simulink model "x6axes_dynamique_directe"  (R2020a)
settings: Solver=VariableStepAuto  StartTime=0.0  StopTime=t(numel(t))  FixedStep=dt  RelTol=1e-3
model workspace: external: MATLAB File (data not in the file)
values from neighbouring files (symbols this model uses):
  D = [10 10 10 0 0 0]    [TP_6Axes_main.m]
  mu = mu/3    [TP_6Axes_main.m]
  P = [10000 10000 10000 1000 1000 1000]    [TP_6Axes_main.m]
  q_targ = zeros(6,numel(X(1,:)))    [TP_6axes_trajectoire_rectangulaire_min_jerk.m]
  X = [X1(:,1:numel(X1(1,:))-1) X2]    [concat_motion.m]    (also in MGD_6axes.m = [T(1:3,4);Euler]; Trace_6axes.m = [0 0 0; Trace_6axes_trajectoire.m = [0 0 0)
undefined symbols (not defined in the file or in its folder): deg, kg, m, mm, N, rad, s, smiData, Y, Z
libraries: sm_lib x37, nesl_utility x22

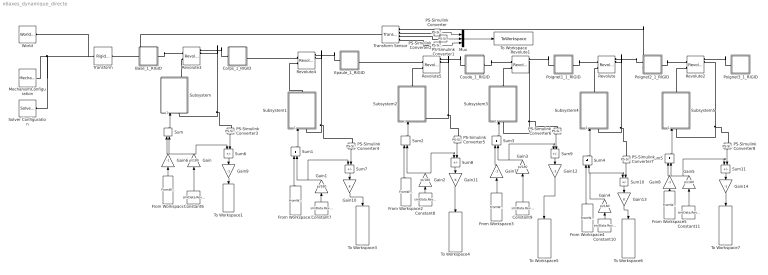
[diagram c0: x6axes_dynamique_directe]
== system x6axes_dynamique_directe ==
  Base_1_RIGID : Subsystem
  Constant10 : Constant  Value=smiData.RevoluteJoint(1).Rz.Pos
  Constant11 : Constant  Value=smiData.RevoluteJoint(3).Rz.Pos
  Constant6 : Constant  Value=smiData.RevoluteJoint(4).Rz.Pos
  Constant7 : Constant  Value=smiData.RevoluteJoint(5).Rz.Pos
  Constant8 : Constant  Value=smiData.RevoluteJoint(6).Rz.Pos
  Constant9 : Constant  Value=smiData.RevoluteJoint(2).Rz.Pos
  Corps_1_RIGID : Subsystem
  Coude_1_RIGID : Subsystem
  Epaule_1_RIGID : Subsystem
  From Workspace : FromWorkspace  VariableName=[t' q_targ(1,:)']
  From Workspace1 : FromWorkspace  VariableName=[t' q_targ(2,:)']
  From Workspace2 : FromWorkspace  VariableName=[t' q_targ(3,:)']
  From Workspace3 : FromWorkspace  VariableName=[t' q_targ(4,:)']
  From Workspace4 : FromWorkspace  VariableName=[t' q_targ(5,:)']
  From Workspace5 : FromWorkspace  VariableName=[t' q_targ(6,:)']
  Gain{,1..5} (6 alike) : Gain  Gain=pi/180
  Gain10 : Gain
  Gain11 : Gain
  Gain{6..9,12,14} (6 alike) : Gain  Gain=-1
  Gain13 : Gain
  MechanismConfiguration : sm_lib/Utilities/Mechanism Configuration  UniformGravity=Constant  GravityVector=[0 0 -9.80665]  GravityUnits=m/s^2  LinearizationDelta=0.001
  Mux : Mux  Inputs=3
  PS-Simulink Converter : nesl_utility/PS-Simulink Converter  PhysicalDomain=network_engine_domain  SubClassName=ps_output  LeftPortType=input  RightPortType=output  PseudoPeriodic=off  Frequencies=[]  Unit=m  AffineConversion=off
  PS-Simulink Converter1 : nesl_utility/PS-Simulink Converter  PhysicalDomain=network_engine_domain  SubClassName=ps_output  LeftPortType=input  RightPortType=output  PseudoPeriodic=off  Frequencies=[]  Unit=m  AffineConversion=off
  PS-Simulink Converter2 : nesl_utility/PS-Simulink Converter  PhysicalDomain=network_engine_domain  SubClassName=ps_output  LeftPortType=input  RightPortType=output  PseudoPeriodic=off  Frequencies=[]  Unit=m  AffineConversion=off
  PS-Simulink Converter{3..8} (6 alike) : nesl_utility/PS-Simulink Converter  PhysicalDomain=network_engine_domain  SubClassName=ps_output  LeftPortType=input  RightPortType=output  PseudoPeriodic=off  Frequencies=[]  Unit=rad  AffineConversion=off
  Poignet1_1_RIGID : Subsystem
  Poignet2_1_RIGID : Subsystem
  Poignet3_1_RIGID : Subsystem
  Revolute : sm_lib/Joints/Revolute Joint  JointMode=Normal  SenseConstraintForce=off  SenseConstraintForceX=off  SenseConstraintForceY=off  SenseConstraintForceZ=off  SenseConstraintTorque=off  SenseConstraintTorqueX=off  SenseConstraintTorqueY=off  SenseConstraintTorqueZ=off  SenseTotalForce=off  SenseTotalForceX=off  SenseTotalForceY=off  SenseTotalForceZ=off  SenseTotalTorque=off  SenseTotalTorqueX=off  SenseTotalTorqueY=off  SenseTotalTorqueZ=off  CompositeWrenchDir=FollowerOnBase  CompositeWrenchFrame=BaseFrame  EquilibriumPosition=0  EquilibriumPositionUnits=rad  SpringStiffness=0  SpringStiffnessUnits=N*m/rad  DampingCoefficient=mu(5)  DampingCoefficientUnits=N*m/(rad/s)  TorqueActuationMode=InputTorque  MotionActuationMode=ComputedMotion  SensePosition=on  SenseVelocity=on  SenseAcceleration=on  SenseTorqueForce=on  SenseLowerLimitTorqueForce=off  SenseUpperLimitTorqueForce=off  LowerLimitSpecify=off  LowerLimitBound=-90  LowerLimitBoundUnits=deg  LowerLimitStiffness=1e4  LowerLimitStiffnessUnits=N*m/deg  LowerLimitDamping=10  LowerLimitDampingUnits=N*m/(deg/s)  LowerLimitTransitionRegionWidth=0.1  LowerLimitTransitionRegionWidthUnits=deg  UpperLimitSpecify=off  UpperLimitBound=90  UpperLimitBoundUnits=deg  UpperLimitStiffness=1e4  UpperLimitStiffnessUnits=N*m/deg  UpperLimitDamping=10  UpperLimitDampingUnits=N*m/(deg/s)  UpperLimitTransitionRegionWidth=0.1  UpperLimitTransitionRegionWidthUnits=deg  PositionTargetSpecify=on  PositionTargetPriority=Low  PositionTargetValue=smiData.RevoluteJoint(1).Rz.Pos*pi/180+q_targ(5,1)  PositionTargetValueUnits=rad  VelocityTargetSpecify=on  VelocityTargetPriority=High  VelocityTargetValue=0  VelocityTargetValueUnits=deg/s
  Revolute1 : sm_lib/Joints/Revolute Joint  JointMode=Normal  SenseConstraintForce=off  SenseConstraintForceX=off  SenseConstraintForceY=off  SenseConstraintForceZ=off  SenseConstraintTorque=off  SenseConstraintTorqueX=off  SenseConstraintTorqueY=off  SenseConstraintTorqueZ=off  SenseTotalForce=off  SenseTotalForceX=off  SenseTotalForceY=off  SenseTotalForceZ=off  SenseTotalTorque=off  SenseTotalTorqueX=off  SenseTotalTorqueY=off  SenseTotalTorqueZ=off  CompositeWrenchDir=FollowerOnBase  CompositeWrenchFrame=BaseFrame  EquilibriumPosition=0  EquilibriumPositionUnits=rad  SpringStiffness=0  SpringStiffnessUnits=N*m/rad  DampingCoefficient=mu(4)  DampingCoefficientUnits=N*m/(rad/s)  TorqueActuationMode=InputTorque  MotionActuationMode=ComputedMotion  SensePosition=on  SenseVelocity=on  SenseAcceleration=on  SenseTorqueForce=on  SenseLowerLimitTorqueForce=off  SenseUpperLimitTorqueForce=off  LowerLimitSpecify=off  LowerLimitBound=-90  LowerLimitBoundUnits=deg  LowerLimitStiffness=1e4  LowerLimitStiffnessUnits=N*m/deg  LowerLimitDamping=10  LowerLimitDampingUnits=N*m/(deg/s)  LowerLimitTransitionRegionWidth=0.1  LowerLimitTransitionRegionWidthUnits=deg  UpperLimitSpecify=off  UpperLimitBound=90  UpperLimitBoundUnits=deg  UpperLimitStiffness=1e4  UpperLimitStiffnessUnits=N*m/deg  UpperLimitDamping=10  UpperLimitDampingUnits=N*m/(deg/s)  UpperLimitTransitionRegionWidth=0.1  UpperLimitTransitionRegionWidthUnits=deg  PositionTargetSpecify=on  PositionTargetPriority=High  PositionTargetValue=smiData.RevoluteJoint(2).Rz.Pos*pi/180-q_targ(4,1)  PositionTargetValueUnits=rad  VelocityTargetSpecify=on  VelocityTargetPriority=High  VelocityTargetValue=0  VelocityTargetValueUnits=deg/s
  Revolute2 : sm_lib/Joints/Revolute Joint  JointMode=Normal  SenseConstraintForce=off  SenseConstraintForceX=off  SenseConstraintForceY=off  SenseConstraintForceZ=off  SenseConstraintTorque=off  SenseConstraintTorqueX=off  SenseConstraintTorqueY=off  SenseConstraintTorqueZ=off  SenseTotalForce=off  SenseTotalForceX=off  SenseTotalForceY=off  SenseTotalForceZ=off  SenseTotalTorque=off  SenseTotalTorqueX=off  SenseTotalTorqueY=off  SenseTotalTorqueZ=off  CompositeWrenchDir=FollowerOnBase  CompositeWrenchFrame=BaseFrame  EquilibriumPosition=0  EquilibriumPositionUnits=rad  SpringStiffness=0  SpringStiffnessUnits=N*m/rad  DampingCoefficient=mu(6)  DampingCoefficientUnits=N*m/(rad/s)  TorqueActuationMode=InputTorque  MotionActuationMode=ComputedMotion  SensePosition=on  SenseVelocity=on  SenseAcceleration=on  SenseTorqueForce=on  SenseLowerLimitTorqueForce=off  SenseUpperLimitTorqueForce=off  LowerLimitSpecify=off  LowerLimitBound=-90  LowerLimitBoundUnits=deg  LowerLimitStiffness=1e4  LowerLimitStiffnessUnits=N*m/deg  LowerLimitDamping=10  LowerLimitDampingUnits=N*m/(deg/s)  LowerLimitTransitionRegionWidth=0.1  LowerLimitTransitionRegionWidthUnits=deg  UpperLimitSpecify=off  UpperLimitBound=90  UpperLimitBoundUnits=deg  UpperLimitStiffness=1e4  UpperLimitStiffnessUnits=N*m/deg  UpperLimitDamping=10  UpperLimitDampingUnits=N*m/(deg/s)  UpperLimitTransitionRegionWidth=0.1  UpperLimitTransitionRegionWidthUnits=deg  PositionTargetSpecify=on  PositionTargetPriority=Low  PositionTargetValue=smiData.RevoluteJoint(3).Rz.Pos*pi/180-q_targ(6,1)  PositionTargetValueUnits=rad  VelocityTargetSpecify=on  VelocityTargetPriority=High  VelocityTargetValue=0  VelocityTargetValueUnits=deg/s
  Revolute3 : sm_lib/Joints/Revolute Joint  JointMode=Normal  SenseConstraintForce=off  SenseConstraintForceX=off  SenseConstraintForceY=off  SenseConstraintForceZ=off  SenseConstraintTorque=off  SenseConstraintTorqueX=off  SenseConstraintTorqueY=off  SenseConstraintTorqueZ=off  SenseTotalForce=off  SenseTotalForceX=off  SenseTotalForceY=off  SenseTotalForceZ=off  SenseTotalTorque=off  SenseTotalTorqueX=off  SenseTotalTorqueY=off  SenseTotalTorqueZ=off  CompositeWrenchDir=FollowerOnBase  CompositeWrenchFrame=BaseFrame  EquilibriumPosition=0  EquilibriumPositionUnits=rad  SpringStiffness=0  SpringStiffnessUnits=N*m/rad  DampingCoefficient=mu(1)  DampingCoefficientUnits=N*m/(rad/s)  TorqueActuationMode=InputTorque  MotionActuationMode=ComputedMotion  SensePosition=on  SenseVelocity=on  SenseAcceleration=on  SenseTorqueForce=on  SenseLowerLimitTorqueForce=off  SenseUpperLimitTorqueForce=off  LowerLimitSpecify=off  LowerLimitBound=-90  LowerLimitBoundUnits=deg  LowerLimitStiffness=1e4  LowerLimitStiffnessUnits=N*m/deg  LowerLimitDamping=10  LowerLimitDampingUnits=N*m/(deg/s)  LowerLimitTransitionRegionWidth=0.1  LowerLimitTransitionRegionWidthUnits=deg  UpperLimitSpecify=off  UpperLimitBound=90  UpperLimitBoundUnits=deg  UpperLimitStiffness=1e4  UpperLimitStiffnessUnits=N*m/deg  UpperLimitDamping=10  UpperLimitDampingUnits=N*m/(deg/s)  UpperLimitTransitionRegionWidth=0.1  UpperLimitTransitionRegionWidthUnits=deg  PositionTargetSpecify=on  PositionTargetPriority=High  PositionTargetValue=smiData.RevoluteJoint(4).Rz.Pos*pi/180-q_targ(1,1)  PositionTargetValueUnits=rad  VelocityTargetSpecify=on  VelocityTargetPriority=High  VelocityTargetValue=0  VelocityTargetValueUnits=deg/s
  Revolute4 : sm_lib/Joints/Revolute Joint  JointMode=Normal  SenseConstraintForce=off  SenseConstraintForceX=off  SenseConstraintForceY=off  SenseConstraintForceZ=off  SenseConstraintTorque=off  SenseConstraintTorqueX=off  SenseConstraintTorqueY=off  SenseConstraintTorqueZ=off  SenseTotalForce=off  SenseTotalForceX=off  SenseTotalForceY=off  SenseTotalForceZ=off  SenseTotalTorque=off  SenseTotalTorqueX=off  SenseTotalTorqueY=off  SenseTotalTorqueZ=off  CompositeWrenchDir=FollowerOnBase  CompositeWrenchFrame=BaseFrame  EquilibriumPosition=0  EquilibriumPositionUnits=rad  SpringStiffness=0  SpringStiffnessUnits=N*m/rad  DampingCoefficient=mu(2)  DampingCoefficientUnits=N*m/(rad/s)  TorqueActuationMode=InputTorque  MotionActuationMode=ComputedMotion  SensePosition=on  SenseVelocity=on  SenseAcceleration=on  SenseTorqueForce=on  SenseLowerLimitTorqueForce=off  SenseUpperLimitTorqueForce=off  LowerLimitSpecify=off  LowerLimitBound=-90  LowerLimitBoundUnits=deg  LowerLimitStiffness=1e4  LowerLimitStiffnessUnits=N*m/deg  LowerLimitDamping=10  LowerLimitDampingUnits=N*m/(deg/s)  LowerLimitTransitionRegionWidth=0.1  LowerLimitTransitionRegionWidthUnits=deg  UpperLimitSpecify=off  UpperLimitBound=90  UpperLimitBoundUnits=deg  UpperLimitStiffness=1e4  UpperLimitStiffnessUnits=N*m/deg  UpperLimitDamping=10  UpperLimitDampingUnits=N*m/(deg/s)  UpperLimitTransitionRegionWidth=0.1  UpperLimitTransitionRegionWidthUnits=deg  PositionTargetSpecify=on  PositionTargetPriority=High  PositionTargetValue=smiData.RevoluteJoint(5).Rz.Pos*pi/180+q_targ(2,1)  PositionTargetValueUnits=rad  VelocityTargetSpecify=on  VelocityTargetPriority=High  VelocityTargetValue=0  VelocityTargetValueUnits=deg/s
  Revolute5 : sm_lib/Joints/Revolute Joint  JointMode=Normal  SenseConstraintForce=off  SenseConstraintForceX=off  SenseConstraintForceY=off  SenseConstraintForceZ=off  SenseConstraintTorque=off  SenseConstraintTorqueX=off  SenseConstraintTorqueY=off  SenseConstraintTorqueZ=off  SenseTotalForce=off  SenseTotalForceX=off  SenseTotalForceY=off  SenseTotalForceZ=off  SenseTotalTorque=off  SenseTotalTorqueX=off  SenseTotalTorqueY=off  SenseTotalTorqueZ=off  CompositeWrenchDir=FollowerOnBase  CompositeWrenchFrame=BaseFrame  EquilibriumPosition=0  EquilibriumPositionUnits=rad  SpringStiffness=0  SpringStiffnessUnits=N*m/rad  DampingCoefficient=mu(3)  DampingCoefficientUnits=N*m/(rad/s)  TorqueActuationMode=InputTorque  MotionActuationMode=ComputedMotion  SensePosition=on  SenseVelocity=on  SenseAcceleration=on  SenseTorqueForce=on  SenseLowerLimitTorqueForce=off  SenseUpperLimitTorqueForce=off  LowerLimitSpecify=off  LowerLimitBound=-90  LowerLimitBoundUnits=deg  LowerLimitStiffness=1e4  LowerLimitStiffnessUnits=N*m/deg  LowerLimitDamping=10  LowerLimitDampingUnits=N*m/(deg/s)  LowerLimitTransitionRegionWidth=0.1  LowerLimitTransitionRegionWidthUnits=deg  UpperLimitSpecify=off  UpperLimitBound=90  UpperLimitBoundUnits=deg  UpperLimitStiffness=1e4  UpperLimitStiffnessUnits=N*m/deg  UpperLimitDamping=10  UpperLimitDampingUnits=N*m/(deg/s)  UpperLimitTransitionRegionWidth=0.1  UpperLimitTransitionRegionWidthUnits=deg  PositionTargetSpecify=on  PositionTargetPriority=High  PositionTargetValue=smiData.RevoluteJoint(6).Rz.Pos*pi/180+q_targ(3,1)  PositionTargetValueUnits=rad  VelocityTargetSpecify=on  VelocityTargetPriority=High  VelocityTargetValue=0  VelocityTargetValueUnits=deg/s
  Solver Configuration : nesl_utility/Solver Configuration  PhysicalDomain=network_engine_domain  SubClassName=solver  LeftPortType=input  RightPortType=generic  Tones=[]  Harmonics=[]  SimulateNoise=off  Profile=off  UseLocalSampling=off  EnableSwitchedLinearOptims=on  FrequencyDomain=off  UseCCode=off  RelTol=0.001  AbsTol=1e-06  MinStep=1e-09  ToWorkspace=off  RevertToSquareIcSolve=off  NumHomotopyIterations=100  PhasorMode=off  PhasorModeNumHarmonics=1  DoDC=off  ResidualTolerance=1e-09  UseLocalSolver=off  LocalSolverChoice=NE_BACKWARD_EULER_ADVANCER  LocalSolverSampleTime=0.001  DoFixedCost=off  MaxNonlinIter=3  MaxModeIter=2  LinearAlgebra=auto  EquationFormulation=NE_TIME_EF  DelaysMemoryBudget=1024  AutomaticFiltering=on  FilteringTimeConstant=0.001  PartitionStorageMethod=AS_NEEDED  PartitionMemoryBudget=1024  PartitionMethod=ROBUST
  Subsystem : Subsystem
  Subsystem1 : Subsystem
  Subsystem2 : Subsystem
  Subsystem3 : Subsystem
  Subsystem4 : Subsystem
  Subsystem5 : Subsystem
  Sum{,1..5} (6 alike) : Sum  Inputs=|++
  Sum{6..11} (6 alike) : Sum  Inputs=|-+
  To Workspace : ToWorkspace  VariableName=position_poignet  SampleTime=-1
  To Workspace1 : ToWorkspace  VariableName=qreal1  SaveFormat=Timeseries  SampleTime=-1
  To Workspace3 : ToWorkspace  VariableName=qreal2  SaveFormat=Timeseries  SampleTime=-1
  To Workspace4 : ToWorkspace  VariableName=qreal3  SaveFormat=Timeseries  SampleTime=-1
  To Workspace5 : ToWorkspace  VariableName=qreal4  SaveFormat=Timeseries  SampleTime=-1
  To Workspace6 : ToWorkspace  VariableName=qreal5  SaveFormat=Timeseries  SampleTime=-1
  To Workspace7 : ToWorkspace  VariableName=qreal6  SaveFormat=Timeseries  SampleTime=-1
  Transform : sm_lib/Frames and Transforms/Rigid Transform  TranslationMethod=Cartesian  TranslationStandardOffset=0  TranslationLengthUnit=mm  TranslationStandardAxis=+Z  TranslationCartesianOffset=smiData.RigidTransform(10).translation  TranslationROffset=0  TranslationROffsetUnits=m  TranslationZOffset=0  TranslationZOffsetUnits=m  TranslationThetaOffset=0  TranslationThetaOffsetUnits=deg  RotationMethod=ArbitraryAxis  RotationAngleUnits=rad  RotationStandardAxis=+Z  RotationAngle=smiData.RigidTransform(10).angle  RotationArbitraryAxis=smiData.RigidTransform(10).axis  FollAlignAxisA=+X  BaseAlignAxisA=+Y  FollAlignAxisB=+Y  BaseAlignAxisB=+Z  RotationSequenceAxes=FollowerAxes  RotationSequence=XYX  RotationSequenceAngles=[0 0 0]  RotationSequenceAnglesUnits=deg  RotationMatrix=[1 0 0; 0 1 0; 0 0 1]
  Transform Sensor : sm_lib/Frames and Transforms/Transform Sensor  MeasurementFrame=World  SenseAngle=off  SenseAxis=off  SenseAngle1=off  SenseAngle2=off  SenseAngle3=off  SenseQ=off  SenseR=off  SenseOmegaX=off  SenseOmegaY=off  SenseOmegaZ=off  SenseOmega1=off  SenseOmega2=off  SenseOmega3=off  SenseQDot=off  SenseRDot=off  SenseAlphaX=off  SenseAlphaY=off  SenseAlphaZ=off  SenseAlpha1=off  SenseAlpha2=off  SenseAlpha3=off  SenseQDDot=off  SenseRDDot=off  SenseX=on  SenseY=on  SenseZ=on  SenseRad=off  SenseAzim=off  SenseDist=off  SenseInc=off  SenseXDot=off  SenseYDot=off  SenseZDot=off  SenseRadDot=off  SenseAzimDot=off  SenseDistDot=off  SenseIncDot=off  SenseXDDot=off  SenseYDDot=off  SenseZDDot=off  SenseRadDDot=off  SenseAzimDDot=off  SenseDistDDot=off  SenseIncDDot=off
  World : sm_lib/Frames and Transforms/World Frame
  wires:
  PS-Simulink Converter/1 -> Mux/1
  PS-Simulink Converter1/1 -> Mux/2
  PS-Simulink Converter2/1 -> Mux/3
  Mux/1 -> To Workspace/1
  From Workspace2/1 -> Sum2/1
  From Workspace1/1 -> Sum1/1
  From Workspace3/1 -> Gain7/1
  From Workspace4/1 -> Sum4/1
  Constant10/1 -> Gain4/1
  Constant11/1 -> Gain5/1
  Constant6/1 -> Gain/1
  Gain8/1 -> Sum5/1
  Constant8/1 -> Gain2/1
  Gain7/1 -> Sum3/1
  Gain6/1 -> Sum/1
  Sum5/1 -> Subsystem5/1(position voulue)
  Sum2/1 -> Subsystem2/1(position voulue)
  Constant7/1 -> Gain1/1
  Gain/1 -> Sum/2, Sum6/1
  Sum1/1 -> Subsystem1/1(position voulue)
  From Workspace/1 -> Gain6/1
  From Workspace5/1 -> Gain8/1
  Sum3/1 -> Subsystem3/1(position voulue)
  Constant9/1 -> Gain3/1
  Sum/1 -> Subsystem/1(position voulue)
  Sum4/1 -> Subsystem4/1(position voulue)
  PS-Simulink Converter3/1 -> Sum6/2
  Sum6/1 -> Gain9/1
  Gain9/1 -> To Workspace1/1
  Gain1/1 -> Sum7/1, Sum1/2
  PS-Simulink Converter4/1 -> Sum7/2
  Sum7/1 -> Gain10/1
  Gain10/1 -> To Workspace3/1
  PS-Simulink Converter5/1 -> Sum8/2
  Gain2/1 -> Sum2/2, Sum8/1
  Gain11/1 -> To Workspace4/1
  Sum8/1 -> Gain11/1
  Gain12/1 -> To Workspace5/1
  Gain3/1 -> Sum9/1, Sum3/2
  PS-Simulink Converter6/1 -> Sum9/2
  Sum9/1 -> Gain12/1
  Gain4/1 -> Sum10/1, Sum4/2
  PS-Simulink Converter7/1 -> Sum10/2
  Sum10/1 -> Gain13/1
  Gain13/1 -> To Workspace6/1
  Gain14/1 -> To Workspace7/1
  Gain5/1 -> Sum11/1, Sum5/2
  PS-Simulink Converter8/1 -> Sum11/2
  Sum11/1 -> Gain14/1
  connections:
  Transform/LConn1 -- MechanismConfiguration/RConn1 -- Solver Configuration/RConn1 -- World/RConn1
  Poignet1_1_RIGID/RConn1 -- Revolute/LConn1
  Corps_1_RIGID/RConn1 -- Revolute4/LConn1
  Epaule_1_RIGID/LConn1 -- Revolute4/RConn1
  Epaule_1_RIGID/RConn1 -- Revolute5/LConn1
  Coude_1_RIGID/LConn1 -- Revolute5/RConn1
  Poignet2_1_RIGID/LConn1 -- Revolute/RConn1
  Coude_1_RIGID/RConn1 -- Revolute1/LConn1
  Poignet1_1_RIGID/LConn1 -- Revolute1/RConn1
  Poignet2_1_RIGID/RConn1 -- Revolute2/LConn1
  Poignet3_1_RIGID/LConn1 -- Revolute2/RConn1
  Base_1_RIGID/RConn1 -- Revolute3/LConn1
  Corps_1_RIGID/LConn1 -- Revolute3/RConn1
  Base_1_RIGID/LConn1 -- Transform Sensor/LConn1 -- Transform/RConn1
  Poignet2_1_RIGID/LConn2 -- Transform Sensor/RConn1
  PS-Simulink Converter/LConn1 -- Transform Sensor/RConn2
  PS-Simulink Converter2/LConn1 -- Transform Sensor/RConn4
  PS-Simulink Converter1/LConn1 -- Transform Sensor/RConn3
  Subsystem/LConn1 -- PS-Simulink Converter3/LConn1 -- Revolute3/RConn2
  Revolute3/LConn2 -- Subsystem/RConn1
  Subsystem1/RConn1 -- Revolute4/LConn2
  Subsystem1/LConn1 -- PS-Simulink Converter4/LConn1 -- Revolute4/RConn2
  Subsystem2/RConn1 -- Revolute5/LConn2
  Subsystem2/LConn1 -- PS-Simulink Converter5/LConn1 -- Revolute5/RConn2
  Subsystem3/RConn1 -- Revolute1/LConn2
  Revolute1/RConn2 -- PS-Simulink Converter6/LConn1 -- Subsystem3/LConn1
  Subsystem4/RConn1 -- Revolute/LConn2
  Subsystem4/LConn1 -- PS-Simulink Converter7/LConn1 -- Revolute/RConn2
  Subsystem5/RConn1 -- Revolute2/LConn2
  Revolute2/RConn2 -- PS-Simulink Converter8/LConn1 -- Subsystem5/LConn1

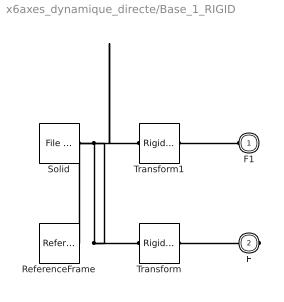
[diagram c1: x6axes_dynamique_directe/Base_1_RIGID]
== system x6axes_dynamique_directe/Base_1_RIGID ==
  ReferenceFrame : sm_lib/Frames and Transforms/Reference Frame
  Solid : sm_lib/Body Elements/File Solid  ExtGeomFileName=Base_Défaut_sldprt.STL  UnitType=Custom  ExtGeomFileUnits=mm  StepReaderType=HEX  ExportConvexHullGeometry=off  InertiaType=Custom  Mass=smiData.Solid(3).mass  MassUnits=kg  CenterOfMass=smiData.Solid(3).CoM  CenterOfMassUnits=mm  MomentsOfInertia=smiData.Solid(3).MoI  MomentsOfInertiaUnits=kg*mm^2  ProductsOfInertia=smiData.Solid(3).PoI  ProductsOfInertiaUnits=kg*mm^2  BasedOnType=DensityFromFile  Density=1000  DensityUnits=kg/m^3  DoExposeReferenceFrame=on  SerializedFrames=<Frames/>  GraphicType=FromGeometry  MarkerShape=Sphere  MarkerSize=10  GraphicVisPropType=SimpleVisualProperties  GraphicDiffuseColor=smiData.Solid(3).color  GraphicSpecularColor=[0.5 0.5 0.5 1.0]  GraphicAmbientColor=[0.15 0.15 0.15 1.0]  GraphicEmissiveColor=[0.0 0.0 0.0 1.0]  GraphicShininess=75  GraphicOpacity=smiData.Solid(3).opacity
  Transform : sm_lib/Frames and Transforms/Rigid Transform  TranslationMethod=Cartesian  TranslationStandardOffset=0  TranslationLengthUnit=mm  TranslationStandardAxis=+Z  TranslationCartesianOffset=smiData.RigidTransform(7).translation  TranslationROffset=0  TranslationROffsetUnits=m  TranslationZOffset=0  TranslationZOffsetUnits=m  TranslationThetaOffset=0  TranslationThetaOffsetUnits=deg  RotationMethod=ArbitraryAxis  RotationAngleUnits=rad  RotationStandardAxis=+Z  RotationAngle=smiData.RigidTransform(7).angle  RotationArbitraryAxis=smiData.RigidTransform(7).axis  FollAlignAxisA=+X  BaseAlignAxisA=+Y  FollAlignAxisB=+Y  BaseAlignAxisB=+Z  RotationSequenceAxes=FollowerAxes  RotationSequence=XYX  RotationSequenceAngles=[0 0 0]  RotationSequenceAnglesUnits=deg  RotationMatrix=[1 0 0; 0 1 0; 0 0 1]
  Transform1 : sm_lib/Frames and Transforms/Rigid Transform  TranslationMethod=Cartesian  TranslationStandardOffset=0  TranslationLengthUnit=mm  TranslationStandardAxis=+Z  TranslationCartesianOffset=smiData.RigidTransform(9).translation  TranslationROffset=0  TranslationROffsetUnits=m  TranslationZOffset=0  TranslationZOffsetUnits=m  TranslationThetaOffset=0  TranslationThetaOffsetUnits=deg  RotationMethod=ArbitraryAxis  RotationAngleUnits=rad  RotationStandardAxis=+Z  RotationAngle=smiData.RigidTransform(9).angle  RotationArbitraryAxis=smiData.RigidTransform(9).axis  FollAlignAxisA=+X  BaseAlignAxisA=+Y  FollAlignAxisB=+Y  BaseAlignAxisB=+Z  RotationSequenceAxes=FollowerAxes  RotationSequence=XYX  RotationSequenceAngles=[0 0 0]  RotationSequenceAnglesUnits=deg  RotationMatrix=[1 0 0; 0 1 0; 0 0 1]
  F1 : PMIOPort  Side=Left
  F : PMIOPort  Port=2  Side=Right
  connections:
  Solid/RConn1 -- ReferenceFrame/RConn1 -- Transform/LConn1 -- Transform1/LConn1
  Transform/RConn1 -- F/RConn1
  Transform1/RConn1 -- F1/RConn1

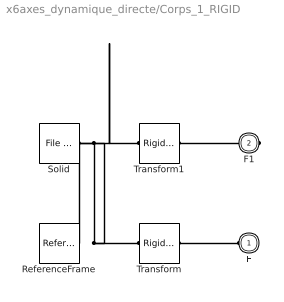
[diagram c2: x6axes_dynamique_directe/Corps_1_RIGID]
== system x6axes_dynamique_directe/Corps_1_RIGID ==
  ReferenceFrame : sm_lib/Frames and Transforms/Reference Frame
  Solid : sm_lib/Body Elements/File Solid  ExtGeomFileName=Corps_Défaut_sldprt.STL  UnitType=Custom  ExtGeomFileUnits=mm  StepReaderType=HEX  ExportConvexHullGeometry=off  InertiaType=Custom  Mass=smiData.Solid(2).mass  MassUnits=kg  CenterOfMass=smiData.Solid(2).CoM  CenterOfMassUnits=mm  MomentsOfInertia=smiData.Solid(2).MoI  MomentsOfInertiaUnits=kg*mm^2  ProductsOfInertia=smiData.Solid(2).PoI  ProductsOfInertiaUnits=kg*mm^2  BasedOnType=DensityFromFile  Density=1000  DensityUnits=kg/m^3  DoExposeReferenceFrame=on  SerializedFrames=<Frames/>  GraphicType=FromGeometry  MarkerShape=Sphere  MarkerSize=10  GraphicVisPropType=SimpleVisualProperties  GraphicDiffuseColor=smiData.Solid(2).color  GraphicSpecularColor=[0.5 0.5 0.5 1.0]  GraphicAmbientColor=[0.15 0.15 0.15 1.0]  GraphicEmissiveColor=[0.0 0.0 0.0 1.0]  GraphicShininess=75  GraphicOpacity=smiData.Solid(2).opacity
  Transform : sm_lib/Frames and Transforms/Rigid Transform  TranslationMethod=Cartesian  TranslationStandardOffset=0  TranslationLengthUnit=mm  TranslationStandardAxis=+Z  TranslationCartesianOffset=smiData.RigidTransform(8).translation  TranslationROffset=0  TranslationROffsetUnits=m  TranslationZOffset=0  TranslationZOffsetUnits=m  TranslationThetaOffset=0  TranslationThetaOffsetUnits=deg  RotationMethod=ArbitraryAxis  RotationAngleUnits=rad  RotationStandardAxis=+Z  RotationAngle=smiData.RigidTransform(8).angle  RotationArbitraryAxis=smiData.RigidTransform(8).axis  FollAlignAxisA=+X  BaseAlignAxisA=+Y  FollAlignAxisB=+Y  BaseAlignAxisB=+Z  RotationSequenceAxes=FollowerAxes  RotationSequence=XYX  RotationSequenceAngles=[0 0 0]  RotationSequenceAnglesUnits=deg  RotationMatrix=[1 0 0; 0 1 0; 0 0 1]
  Transform1 : sm_lib/Frames and Transforms/Rigid Transform  TranslationMethod=Cartesian  TranslationStandardOffset=0  TranslationLengthUnit=mm  TranslationStandardAxis=+Z  TranslationCartesianOffset=smiData.RigidTransform(11).translation  TranslationROffset=0  TranslationROffsetUnits=m  TranslationZOffset=0  TranslationZOffsetUnits=m  TranslationThetaOffset=0  TranslationThetaOffsetUnits=deg  RotationMethod=ArbitraryAxis  RotationAngleUnits=rad  RotationStandardAxis=+Z  RotationAngle=smiData.RigidTransform(11).angle  RotationArbitraryAxis=smiData.RigidTransform(11).axis  FollAlignAxisA=+X  BaseAlignAxisA=+Y  FollAlignAxisB=+Y  BaseAlignAxisB=+Z  RotationSequenceAxes=FollowerAxes  RotationSequence=XYX  RotationSequenceAngles=[0 0 0]  RotationSequenceAnglesUnits=deg  RotationMatrix=[1 0 0; 0 1 0; 0 0 1]
  F : PMIOPort  Side=Left
  F1 : PMIOPort  Port=2  Side=Right
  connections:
  Solid/RConn1 -- ReferenceFrame/RConn1 -- Transform/LConn1 -- Transform1/LConn1
  Transform/RConn1 -- F/RConn1
  Transform1/RConn1 -- F1/RConn1

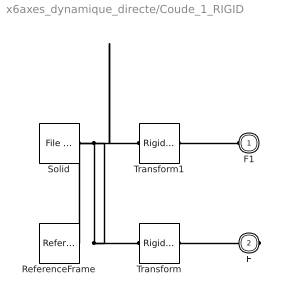
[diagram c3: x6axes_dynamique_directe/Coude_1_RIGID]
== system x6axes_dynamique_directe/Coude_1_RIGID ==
  ReferenceFrame : sm_lib/Frames and Transforms/Reference Frame
  Solid : sm_lib/Body Elements/File Solid  ExtGeomFileName=Coude_Défaut_sldprt.STL  UnitType=Custom  ExtGeomFileUnits=mm  StepReaderType=HEX  ExportConvexHullGeometry=off  InertiaType=Custom  Mass=smiData.Solid(5).mass  MassUnits=kg  CenterOfMass=smiData.Solid(5).CoM  CenterOfMassUnits=mm  MomentsOfInertia=smiData.Solid(5).MoI  MomentsOfInertiaUnits=kg*mm^2  ProductsOfInertia=smiData.Solid(5).PoI  ProductsOfInertiaUnits=kg*mm^2  BasedOnType=DensityFromFile  Density=1000  DensityUnits=kg/m^3  DoExposeReferenceFrame=on  SerializedFrames=<Frames/>  GraphicType=FromGeometry  MarkerShape=Sphere  MarkerSize=10  GraphicVisPropType=SimpleVisualProperties  GraphicDiffuseColor=smiData.Solid(5).color  GraphicSpecularColor=[0.5 0.5 0.5 1.0]  GraphicAmbientColor=[0.15 0.15 0.15 1.0]  GraphicEmissiveColor=[0.0 0.0 0.0 1.0]  GraphicShininess=75  GraphicOpacity=smiData.Solid(5).opacity
  Transform : sm_lib/Frames and Transforms/Rigid Transform  TranslationMethod=Cartesian  TranslationStandardOffset=0  TranslationLengthUnit=mm  TranslationStandardAxis=+Z  TranslationCartesianOffset=smiData.RigidTransform(3).translation  TranslationROffset=0  TranslationROffsetUnits=m  TranslationZOffset=0  TranslationZOffsetUnits=m  TranslationThetaOffset=0  TranslationThetaOffsetUnits=deg  RotationMethod=ArbitraryAxis  RotationAngleUnits=rad  RotationStandardAxis=+Z  RotationAngle=smiData.RigidTransform(3).angle  RotationArbitraryAxis=smiData.RigidTransform(3).axis  FollAlignAxisA=+X  BaseAlignAxisA=+Y  FollAlignAxisB=+Y  BaseAlignAxisB=+Z  RotationSequenceAxes=FollowerAxes  RotationSequence=XYX  RotationSequenceAngles=[0 0 0]  RotationSequenceAnglesUnits=deg  RotationMatrix=[1 0 0; 0 1 0; 0 0 1]
  Transform1 : sm_lib/Frames and Transforms/Rigid Transform  TranslationMethod=Cartesian  TranslationStandardOffset=0  TranslationLengthUnit=mm  TranslationStandardAxis=+Z  TranslationCartesianOffset=smiData.RigidTransform(14).translation  TranslationROffset=0  TranslationROffsetUnits=m  TranslationZOffset=0  TranslationZOffsetUnits=m  TranslationThetaOffset=0  TranslationThetaOffsetUnits=deg  RotationMethod=ArbitraryAxis  RotationAngleUnits=rad  RotationStandardAxis=+Z  RotationAngle=smiData.RigidTransform(14).angle  RotationArbitraryAxis=smiData.RigidTransform(14).axis  FollAlignAxisA=+X  BaseAlignAxisA=+Y  FollAlignAxisB=+Y  BaseAlignAxisB=+Z  RotationSequenceAxes=FollowerAxes  RotationSequence=XYX  RotationSequenceAngles=[0 0 0]  RotationSequenceAnglesUnits=deg  RotationMatrix=[1 0 0; 0 1 0; 0 0 1]
  F1 : PMIOPort  Side=Left
  F : PMIOPort  Port=2  Side=Right
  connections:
  Solid/RConn1 -- ReferenceFrame/RConn1 -- Transform/LConn1 -- Transform1/LConn1
  Transform/RConn1 -- F/RConn1
  Transform1/RConn1 -- F1/RConn1

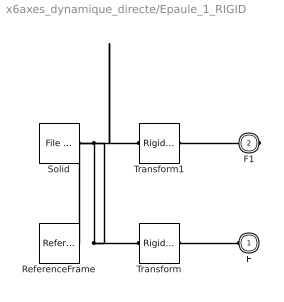
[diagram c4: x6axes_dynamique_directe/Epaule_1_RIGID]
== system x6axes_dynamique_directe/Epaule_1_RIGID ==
  ReferenceFrame : sm_lib/Frames and Transforms/Reference Frame
  Solid : sm_lib/Body Elements/File Solid  ExtGeomFileName=Epaule_Défaut_sldprt.STL  UnitType=Custom  ExtGeomFileUnits=mm  StepReaderType=HEX  ExportConvexHullGeometry=off  InertiaType=Custom  Mass=smiData.Solid(7).mass  MassUnits=kg  CenterOfMass=smiData.Solid(7).CoM  CenterOfMassUnits=mm  MomentsOfInertia=smiData.Solid(7).MoI  MomentsOfInertiaUnits=kg*mm^2  ProductsOfInertia=smiData.Solid(7).PoI  ProductsOfInertiaUnits=kg*mm^2  BasedOnType=DensityFromFile  Density=1000  DensityUnits=kg/m^3  DoExposeReferenceFrame=on  SerializedFrames=<Frames/>  GraphicType=FromGeometry  MarkerShape=Sphere  MarkerSize=10  GraphicVisPropType=SimpleVisualProperties  GraphicDiffuseColor=smiData.Solid(7).color  GraphicSpecularColor=[0.5 0.5 0.5 1.0]  GraphicAmbientColor=[0.15 0.15 0.15 1.0]  GraphicEmissiveColor=[0.0 0.0 0.0 1.0]  GraphicShininess=75  GraphicOpacity=smiData.Solid(7).opacity
  Transform : sm_lib/Frames and Transforms/Rigid Transform  TranslationMethod=Cartesian  TranslationStandardOffset=0  TranslationLengthUnit=mm  TranslationStandardAxis=+Z  TranslationCartesianOffset=smiData.RigidTransform(12).translation  TranslationROffset=0  TranslationROffsetUnits=m  TranslationZOffset=0  TranslationZOffsetUnits=m  TranslationThetaOffset=0  TranslationThetaOffsetUnits=deg  RotationMethod=ArbitraryAxis  RotationAngleUnits=rad  RotationStandardAxis=+Z  RotationAngle=smiData.RigidTransform(12).angle  RotationArbitraryAxis=smiData.RigidTransform(12).axis  FollAlignAxisA=+X  BaseAlignAxisA=+Y  FollAlignAxisB=+Y  BaseAlignAxisB=+Z  RotationSequenceAxes=FollowerAxes  RotationSequence=XYX  RotationSequenceAngles=[0 0 0]  RotationSequenceAnglesUnits=deg  RotationMatrix=[1 0 0; 0 1 0; 0 0 1]
  Transform1 : sm_lib/Frames and Transforms/Rigid Transform  TranslationMethod=Cartesian  TranslationStandardOffset=0  TranslationLengthUnit=mm  TranslationStandardAxis=+Z  TranslationCartesianOffset=smiData.RigidTransform(13).translation  TranslationROffset=0  TranslationROffsetUnits=m  TranslationZOffset=0  TranslationZOffsetUnits=m  TranslationThetaOffset=0  TranslationThetaOffsetUnits=deg  RotationMethod=ArbitraryAxis  RotationAngleUnits=rad  RotationStandardAxis=+Z  RotationAngle=smiData.RigidTransform(13).angle  RotationArbitraryAxis=smiData.RigidTransform(13).axis  FollAlignAxisA=+X  BaseAlignAxisA=+Y  FollAlignAxisB=+Y  BaseAlignAxisB=+Z  RotationSequenceAxes=FollowerAxes  RotationSequence=XYX  RotationSequenceAngles=[0 0 0]  RotationSequenceAnglesUnits=deg  RotationMatrix=[1 0 0; 0 1 0; 0 0 1]
  F : PMIOPort  Side=Left
  F1 : PMIOPort  Port=2  Side=Right
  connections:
  Solid/RConn1 -- ReferenceFrame/RConn1 -- Transform/LConn1 -- Transform1/LConn1
  Transform/RConn1 -- F/RConn1
  Transform1/RConn1 -- F1/RConn1

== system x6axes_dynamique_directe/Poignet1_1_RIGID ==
  ReferenceFrame : sm_lib/Frames and Transforms/Reference Frame
  Solid : sm_lib/Body Elements/File Solid  ExtGeomFileName=Poignet1_Défaut_sldprt.STL  UnitType=Custom  ExtGeomFileUnits=mm  StepReaderType=HEX  ExportConvexHullGeometry=off  InertiaType=Custom  Mass=smiData.Solid(6).mass  MassUnits=kg  CenterOfMass=smiData.Solid(6).CoM  CenterOfMassUnits=mm  MomentsOfInertia=smiData.Solid(6).MoI  MomentsOfInertiaUnits=kg*mm^2  ProductsOfInertia=smiData.Solid(6).PoI  ProductsOfInertiaUnits=kg*mm^2  BasedOnType=DensityFromFile  Density=1000  DensityUnits=kg/m^3  DoExposeReferenceFrame=on  SerializedFrames=<Frames/>  GraphicType=FromGeometry  MarkerShape=Sphere  MarkerSize=10  GraphicVisPropType=SimpleVisualProperties  GraphicDiffuseColor=smiData.Solid(6).color  GraphicSpecularColor=[0.5 0.5 0.5 1.0]  GraphicAmbientColor=[0.15 0.15 0.15 1.0]  GraphicEmissiveColor=[0.0 0.0 0.0 1.0]  GraphicShininess=75  GraphicOpacity=smiData.Solid(6).opacity
  Transform : sm_lib/Frames and Transforms/Rigid Transform  TranslationMethod=Cartesian  TranslationStandardOffset=0  TranslationLengthUnit=mm  TranslationStandardAxis=+Z  TranslationCartesianOffset=smiData.RigidTransform(1).translation  TranslationROffset=0  TranslationROffsetUnits=m  TranslationZOffset=0  TranslationZOffsetUnits=m  TranslationThetaOffset=0  TranslationThetaOffsetUnits=deg  RotationMethod=ArbitraryAxis  RotationAngleUnits=rad  RotationStandardAxis=+Z  RotationAngle=smiData.RigidTransform(1).angle  RotationArbitraryAxis=smiData.RigidTransform(1).axis  FollAlignAxisA=+X  BaseAlignAxisA=+Y  FollAlignAxisB=+Y  BaseAlignAxisB=+Z  RotationSequenceAxes=FollowerAxes  RotationSequence=XYX  RotationSequenceAngles=[0 0 0]  RotationSequenceAnglesUnits=deg  RotationMatrix=[1 0 0; 0 1 0; 0 0 1]
  Transform1 : sm_lib/Frames and Transforms/Rigid Transform  TranslationMethod=Cartesian  TranslationStandardOffset=0  TranslationLengthUnit=mm  TranslationStandardAxis=+Z  TranslationCartesianOffset=smiData.RigidTransform(4).translation  TranslationROffset=0  TranslationROffsetUnits=m  TranslationZOffset=0  TranslationZOffsetUnits=m  TranslationThetaOffset=0  TranslationThetaOffsetUnits=deg  RotationMethod=ArbitraryAxis  RotationAngleUnits=rad  RotationStandardAxis=+Z  RotationAngle=smiData.RigidTransform(4).angle  RotationArbitraryAxis=smiData.RigidTransform(4).axis  FollAlignAxisA=+X  BaseAlignAxisA=+Y  FollAlignAxisB=+Y  BaseAlignAxisB=+Z  RotationSequenceAxes=FollowerAxes  RotationSequence=XYX  RotationSequenceAngles=[0 0 0]  RotationSequenceAnglesUnits=deg  RotationMatrix=[1 0 0; 0 1 0; 0 0 1]
  F1 : PMIOPort  Side=Left
  F : PMIOPort  Port=2  Side=Right
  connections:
  Solid/RConn1 -- ReferenceFrame/RConn1 -- Transform/LConn1 -- Transform1/LConn1
  Transform/RConn1 -- F/RConn1
  Transform1/RConn1 -- F1/RConn1

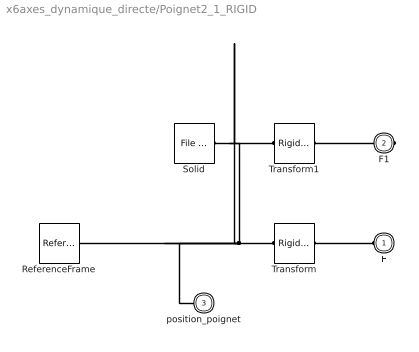
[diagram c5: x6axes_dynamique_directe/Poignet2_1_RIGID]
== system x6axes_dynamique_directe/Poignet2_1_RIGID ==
  ReferenceFrame : sm_lib/Frames and Transforms/Reference Frame
  Solid : sm_lib/Body Elements/File Solid  ExtGeomFileName=Poignet2_Défaut_sldprt.STL  UnitType=Custom  ExtGeomFileUnits=mm  StepReaderType=HEX  ExportConvexHullGeometry=off  InertiaType=Custom  Mass=smiData.Solid(1).mass  MassUnits=kg  CenterOfMass=smiData.Solid(1).CoM  CenterOfMassUnits=mm  MomentsOfInertia=smiData.Solid(1).MoI  MomentsOfInertiaUnits=kg*mm^2  ProductsOfInertia=smiData.Solid(1).PoI  ProductsOfInertiaUnits=kg*mm^2  BasedOnType=DensityFromFile  Density=1000  DensityUnits=kg/m^3  DoExposeReferenceFrame=on  SerializedFrames=<Frames/>  GraphicType=FromGeometry  MarkerShape=Sphere  MarkerSize=10  GraphicVisPropType=SimpleVisualProperties  GraphicDiffuseColor=smiData.Solid(1).color  GraphicSpecularColor=[0.5 0.5 0.5 1.0]  GraphicAmbientColor=[0.15 0.15 0.15 1.0]  GraphicEmissiveColor=[0.0 0.0 0.0 1.0]  GraphicShininess=75  GraphicOpacity=smiData.Solid(1).opacity
  Transform : sm_lib/Frames and Transforms/Rigid Transform  TranslationMethod=Cartesian  TranslationStandardOffset=0  TranslationLengthUnit=mm  TranslationStandardAxis=+Z  TranslationCartesianOffset=smiData.RigidTransform(2).translation  TranslationROffset=0  TranslationROffsetUnits=m  TranslationZOffset=0  TranslationZOffsetUnits=m  TranslationThetaOffset=0  TranslationThetaOffsetUnits=deg  RotationMethod=ArbitraryAxis  RotationAngleUnits=rad  RotationStandardAxis=+Z  RotationAngle=smiData.RigidTransform(2).angle  RotationArbitraryAxis=smiData.RigidTransform(2).axis  FollAlignAxisA=+X  BaseAlignAxisA=+Y  FollAlignAxisB=+Y  BaseAlignAxisB=+Z  RotationSequenceAxes=FollowerAxes  RotationSequence=XYX  RotationSequenceAngles=[0 0 0]  RotationSequenceAnglesUnits=deg  RotationMatrix=[1 0 0; 0 1 0; 0 0 1]
  Transform1 : sm_lib/Frames and Transforms/Rigid Transform  TranslationMethod=Cartesian  TranslationStandardOffset=0  TranslationLengthUnit=mm  TranslationStandardAxis=+Z  TranslationCartesianOffset=smiData.RigidTransform(5).translation  TranslationROffset=0  TranslationROffsetUnits=m  TranslationZOffset=0  TranslationZOffsetUnits=m  TranslationThetaOffset=0  TranslationThetaOffsetUnits=deg  RotationMethod=ArbitraryAxis  RotationAngleUnits=rad  RotationStandardAxis=+Z  RotationAngle=smiData.RigidTransform(5).angle  RotationArbitraryAxis=smiData.RigidTransform(5).axis  FollAlignAxisA=+X  BaseAlignAxisA=+Y  FollAlignAxisB=+Y  BaseAlignAxisB=+Z  RotationSequenceAxes=FollowerAxes  RotationSequence=XYX  RotationSequenceAngles=[0 0 0]  RotationSequenceAnglesUnits=deg  RotationMatrix=[1 0 0; 0 1 0; 0 0 1]
  F : PMIOPort  Side=Left
  F1 : PMIOPort  Port=2  Side=Right
  position_poignet : PMIOPort  Port=3  Side=Left
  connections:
  Solid/RConn1 -- position_poignet/RConn1 -- ReferenceFrame/RConn1 -- Transform/LConn1 -- Transform1/LConn1
  Transform/RConn1 -- F/RConn1
  Transform1/RConn1 -- F1/RConn1

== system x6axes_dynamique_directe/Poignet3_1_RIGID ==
  ReferenceFrame : sm_lib/Frames and Transforms/Reference Frame
  Solid : sm_lib/Body Elements/File Solid  ExtGeomFileName=Poignet3_Défaut_sldprt.STL  UnitType=Custom  ExtGeomFileUnits=mm  StepReaderType=HEX  ExportConvexHullGeometry=off  InertiaType=Custom  Mass=smiData.Solid(4).mass  MassUnits=kg  CenterOfMass=smiData.Solid(4).CoM  CenterOfMassUnits=mm  MomentsOfInertia=smiData.Solid(4).MoI  MomentsOfInertiaUnits=kg*mm^2  ProductsOfInertia=smiData.Solid(4).PoI  ProductsOfInertiaUnits=kg*mm^2  BasedOnType=DensityFromFile  Density=1000  DensityUnits=kg/m^3  DoExposeReferenceFrame=on  SerializedFrames=<Frames/>  GraphicType=FromGeometry  MarkerShape=Sphere  MarkerSize=10  GraphicVisPropType=SimpleVisualProperties  GraphicDiffuseColor=smiData.Solid(4).color  GraphicSpecularColor=[0.5 0.5 0.5 1.0]  GraphicAmbientColor=[0.15 0.15 0.15 1.0]  GraphicEmissiveColor=[0.0 0.0 0.0 1.0]  GraphicShininess=75  GraphicOpacity=smiData.Solid(4).opacity
  Transform : sm_lib/Frames and Transforms/Rigid Transform  TranslationMethod=Cartesian  TranslationStandardOffset=0  TranslationLengthUnit=mm  TranslationStandardAxis=+Z  TranslationCartesianOffset=smiData.RigidTransform(6).translation  TranslationROffset=0  TranslationROffsetUnits=m  TranslationZOffset=0  TranslationZOffsetUnits=m  TranslationThetaOffset=0  TranslationThetaOffsetUnits=deg  RotationMethod=ArbitraryAxis  RotationAngleUnits=rad  RotationStandardAxis=+Z  RotationAngle=smiData.RigidTransform(6).angle  RotationArbitraryAxis=smiData.RigidTransform(6).axis  FollAlignAxisA=+X  BaseAlignAxisA=+Y  FollAlignAxisB=+Y  BaseAlignAxisB=+Z  RotationSequenceAxes=FollowerAxes  RotationSequence=XYX  RotationSequenceAngles=[0 0 0]  RotationSequenceAnglesUnits=deg  RotationMatrix=[1 0 0; 0 1 0; 0 0 1]
  F : PMIOPort  Side=Left
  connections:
  Solid/RConn1 -- ReferenceFrame/RConn1 -- Transform/LConn1
  Transform/RConn1 -- F/RConn1

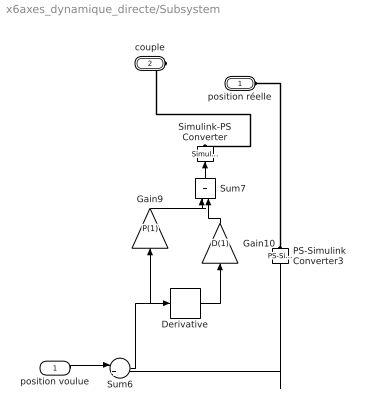
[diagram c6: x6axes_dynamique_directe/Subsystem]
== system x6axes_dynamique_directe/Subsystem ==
  position voulue : Inport
  Derivative : Derivative
  Gain10 : Gain  Gain=D(1)
  Gain9 : Gain  Gain=P(1)
  PS-Simulink Converter3 : nesl_utility/PS-Simulink Converter  PhysicalDomain=network_engine_domain  SubClassName=ps_output  LeftPortType=input  RightPortType=output  PseudoPeriodic=off  Frequencies=[]  Unit=rad  AffineConversion=off
  Simulink-PS Converter : nesl_utility/Simulink-PS Converter  PhysicalDomain=network_engine_domain  SubClassName=ps_input  LeftPortType=input  RightPortType=output  PseudoPeriodic=off  Frequencies=[]  NoiseDistribution=none  NoiseParameters=[]  Unit=N*m  AffineConversion=off  FilteringAndDerivatives=provide  SimscapeFilterOrder=1  InputFilterTimeConstant=0.001  UdotUserProvided=0
  Sum6 : Sum  Inputs=|+-
  Sum7 : Sum  Inputs=|++
  position réelle : PMIOPort  Side=Left
  couple : PMIOPort  Port=2  Side=Right
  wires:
  PS-Simulink Converter3/1 -> Sum6/2
  Gain9/1 -> Sum7/1
  Sum7/1 -> Simulink-PS Converter/1
  Sum6/1 -> Gain9/1, Derivative/1
  Gain10/1 -> Sum7/2
  Derivative/1 -> Gain10/1
  position voulue/1 -> Sum6/1
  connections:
  couple/RConn1 -- Simulink-PS Converter/RConn1
  PS-Simulink Converter3/LConn1 -- position réelle/RConn1

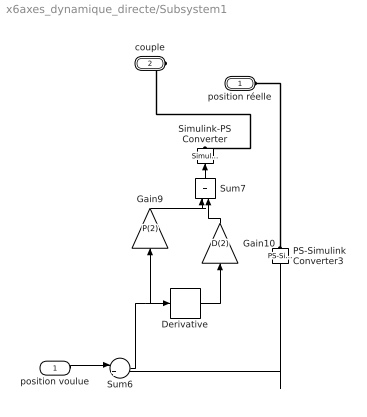
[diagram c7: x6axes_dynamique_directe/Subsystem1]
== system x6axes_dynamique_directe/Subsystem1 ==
  position voulue : Inport
  Derivative : Derivative
  Gain10 : Gain  Gain=D(2)
  Gain9 : Gain  Gain=P(2)
  PS-Simulink Converter3 : nesl_utility/PS-Simulink Converter  PhysicalDomain=network_engine_domain  SubClassName=ps_output  LeftPortType=input  RightPortType=output  PseudoPeriodic=off  Frequencies=[]  Unit=rad  AffineConversion=off
  Simulink-PS Converter : nesl_utility/Simulink-PS Converter  PhysicalDomain=network_engine_domain  SubClassName=ps_input  LeftPortType=input  RightPortType=output  PseudoPeriodic=off  Frequencies=[]  NoiseDistribution=none  NoiseParameters=[]  Unit=N*m  AffineConversion=off  FilteringAndDerivatives=provide  SimscapeFilterOrder=1  InputFilterTimeConstant=0.001  UdotUserProvided=0
  Sum6 : Sum  Inputs=|+-
  Sum7 : Sum  Inputs=|++
  position réelle : PMIOPort  Side=Left
  couple : PMIOPort  Port=2  Side=Right
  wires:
  PS-Simulink Converter3/1 -> Sum6/2
  Gain9/1 -> Sum7/1
  Sum7/1 -> Simulink-PS Converter/1
  Sum6/1 -> Gain9/1, Derivative/1
  Gain10/1 -> Sum7/2
  Derivative/1 -> Gain10/1
  position voulue/1 -> Sum6/1
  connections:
  couple/RConn1 -- Simulink-PS Converter/RConn1
  PS-Simulink Converter3/LConn1 -- position réelle/RConn1

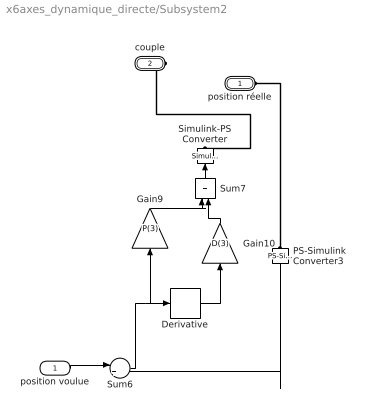
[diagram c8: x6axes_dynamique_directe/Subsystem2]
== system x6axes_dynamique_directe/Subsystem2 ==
  position voulue : Inport
  Derivative : Derivative
  Gain10 : Gain  Gain=D(3)
  Gain9 : Gain  Gain=P(3)
  PS-Simulink Converter3 : nesl_utility/PS-Simulink Converter  PhysicalDomain=network_engine_domain  SubClassName=ps_output  LeftPortType=input  RightPortType=output  PseudoPeriodic=off  Frequencies=[]  Unit=rad  AffineConversion=off
  Simulink-PS Converter : nesl_utility/Simulink-PS Converter  PhysicalDomain=network_engine_domain  SubClassName=ps_input  LeftPortType=input  RightPortType=output  PseudoPeriodic=off  Frequencies=[]  NoiseDistribution=none  NoiseParameters=[]  Unit=N*m  AffineConversion=off  FilteringAndDerivatives=provide  SimscapeFilterOrder=1  InputFilterTimeConstant=0.001  UdotUserProvided=0
  Sum6 : Sum  Inputs=|+-
  Sum7 : Sum  Inputs=|++
  position réelle : PMIOPort  Side=Left
  couple : PMIOPort  Port=2  Side=Right
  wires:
  PS-Simulink Converter3/1 -> Sum6/2
  Gain9/1 -> Sum7/1
  Sum7/1 -> Simulink-PS Converter/1
  Sum6/1 -> Gain9/1, Derivative/1
  Gain10/1 -> Sum7/2
  Derivative/1 -> Gain10/1
  position voulue/1 -> Sum6/1
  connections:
  couple/RConn1 -- Simulink-PS Converter/RConn1
  PS-Simulink Converter3/LConn1 -- position réelle/RConn1

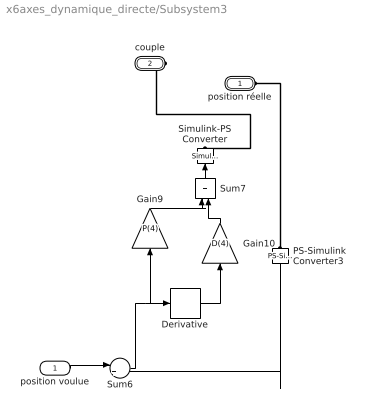
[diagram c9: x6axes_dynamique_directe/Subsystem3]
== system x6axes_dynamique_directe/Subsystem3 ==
  position voulue : Inport
  Derivative : Derivative
  Gain10 : Gain  Gain=D(4)
  Gain9 : Gain  Gain=P(4)
  PS-Simulink Converter3 : nesl_utility/PS-Simulink Converter  PhysicalDomain=network_engine_domain  SubClassName=ps_output  LeftPortType=input  RightPortType=output  PseudoPeriodic=off  Frequencies=[]  Unit=rad  AffineConversion=off
  Simulink-PS Converter : nesl_utility/Simulink-PS Converter  PhysicalDomain=network_engine_domain  SubClassName=ps_input  LeftPortType=input  RightPortType=output  PseudoPeriodic=off  Frequencies=[]  NoiseDistribution=none  NoiseParameters=[]  Unit=N*m  AffineConversion=off  FilteringAndDerivatives=provide  SimscapeFilterOrder=1  InputFilterTimeConstant=0.001  UdotUserProvided=0
  Sum6 : Sum  Inputs=|+-
  Sum7 : Sum  Inputs=|++
  position réelle : PMIOPort  Side=Left
  couple : PMIOPort  Port=2  Side=Right
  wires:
  PS-Simulink Converter3/1 -> Sum6/2
  Gain9/1 -> Sum7/1
  Sum7/1 -> Simulink-PS Converter/1
  Sum6/1 -> Gain9/1, Derivative/1
  Gain10/1 -> Sum7/2
  Derivative/1 -> Gain10/1
  position voulue/1 -> Sum6/1
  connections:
  couple/RConn1 -- Simulink-PS Converter/RConn1
  PS-Simulink Converter3/LConn1 -- position réelle/RConn1

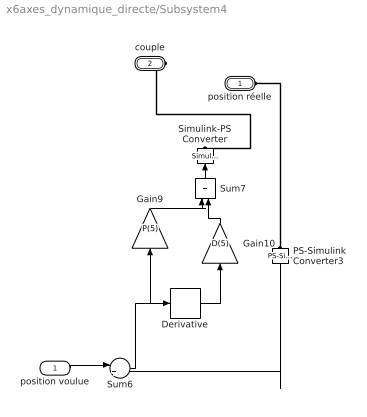
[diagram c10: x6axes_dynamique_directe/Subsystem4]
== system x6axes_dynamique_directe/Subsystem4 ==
  position voulue : Inport
  Derivative : Derivative
  Gain10 : Gain  Gain=D(5)
  Gain9 : Gain  Gain=P(5)
  PS-Simulink Converter3 : nesl_utility/PS-Simulink Converter  PhysicalDomain=network_engine_domain  SubClassName=ps_output  LeftPortType=input  RightPortType=output  PseudoPeriodic=off  Frequencies=[]  Unit=rad  AffineConversion=off
  Simulink-PS Converter : nesl_utility/Simulink-PS Converter  PhysicalDomain=network_engine_domain  SubClassName=ps_input  LeftPortType=input  RightPortType=output  PseudoPeriodic=off  Frequencies=[]  NoiseDistribution=none  NoiseParameters=[]  Unit=N*m  AffineConversion=off  FilteringAndDerivatives=provide  SimscapeFilterOrder=1  InputFilterTimeConstant=0.001  UdotUserProvided=0
  Sum6 : Sum  Inputs=|+-
  Sum7 : Sum  Inputs=|++
  position réelle : PMIOPort  Side=Left
  couple : PMIOPort  Port=2  Side=Right
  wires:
  PS-Simulink Converter3/1 -> Sum6/2
  Gain9/1 -> Sum7/1
  Sum7/1 -> Simulink-PS Converter/1
  Sum6/1 -> Gain9/1, Derivative/1
  Gain10/1 -> Sum7/2
  Derivative/1 -> Gain10/1
  position voulue/1 -> Sum6/1
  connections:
  couple/RConn1 -- Simulink-PS Converter/RConn1
  PS-Simulink Converter3/LConn1 -- position réelle/RConn1

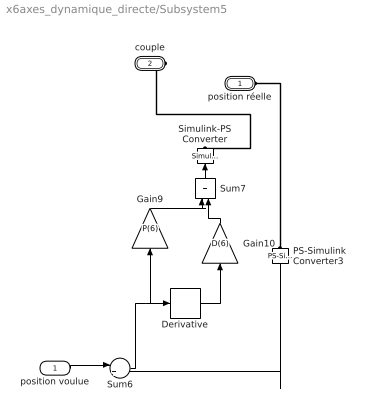
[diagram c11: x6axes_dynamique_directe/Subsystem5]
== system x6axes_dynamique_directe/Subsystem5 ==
  position voulue : Inport
  Derivative : Derivative
  Gain10 : Gain  Gain=D(6)
  Gain9 : Gain  Gain=P(6)
  PS-Simulink Converter3 : nesl_utility/PS-Simulink Converter  PhysicalDomain=network_engine_domain  SubClassName=ps_output  LeftPortType=input  RightPortType=output  PseudoPeriodic=off  Frequencies=[]  Unit=rad  AffineConversion=off
  Simulink-PS Converter : nesl_utility/Simulink-PS Converter  PhysicalDomain=network_engine_domain  SubClassName=ps_input  LeftPortType=input  RightPortType=output  PseudoPeriodic=off  Frequencies=[]  NoiseDistribution=none  NoiseParameters=[]  Unit=N*m  AffineConversion=off  FilteringAndDerivatives=provide  SimscapeFilterOrder=1  InputFilterTimeConstant=0.001  UdotUserProvided=0
  Sum6 : Sum  Inputs=|+-
  Sum7 : Sum  Inputs=|++
  position réelle : PMIOPort  Side=Left
  couple : PMIOPort  Port=2  Side=Right
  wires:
  PS-Simulink Converter3/1 -> Sum6/2
  Gain9/1 -> Sum7/1
  Sum7/1 -> Simulink-PS Converter/1
  Sum6/1 -> Gain9/1, Derivative/1
  Gain10/1 -> Sum7/2
  Derivative/1 -> Gain10/1
  position voulue/1 -> Sum6/1
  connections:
  couple/RConn1 -- Simulink-PS Converter/RConn1
  PS-Simulink Converter3/LConn1 -- position réelle/RConn1
